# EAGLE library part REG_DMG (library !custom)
Regulator of some sort for the DMG screen. Wouldn’t know what it was called if it weren’t for it being written on the part.
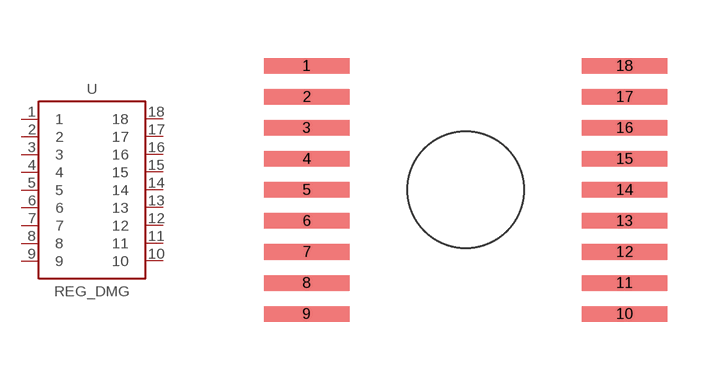
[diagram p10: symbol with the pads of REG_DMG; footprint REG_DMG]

Designator prefix U

## REG_DMG  [REG_DMG]
1  1  pas
2  2  pas
3  3  pas
4  4  pas
5  5  pas
6  6  pas
7  7  pas
8  8  pas
9  9  pas
10  10  pas
11  11  pas
12  12  pas
13  13  pas
14  14  pas
15  15  pas
16  16  pas
17  17  pas
18  18  pas

## Footprint REG_DMG (pad centres in mm)
smd 2.2 x 0.4: 1 -4.1,3.2; 2 -4.1,2.4; 3 -4.1,1.6; 4 -4.1,0.8; 5 -4.1,0; 6 -4.1,-0.8; 7 -4.1,-1.6; 8 -4.1,-2.4; 9 -4.1,-3.2; 10 4.1,-3.2; 11 4.1,-2.4; 12 4.1,-1.6; 13 4.1,-0.8; 14 4.1,0; 15 4.1,0.8; 16 4.1,1.6; 17 4.1,2.4; 18 4.1,3.2
hole 3 at 0,0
